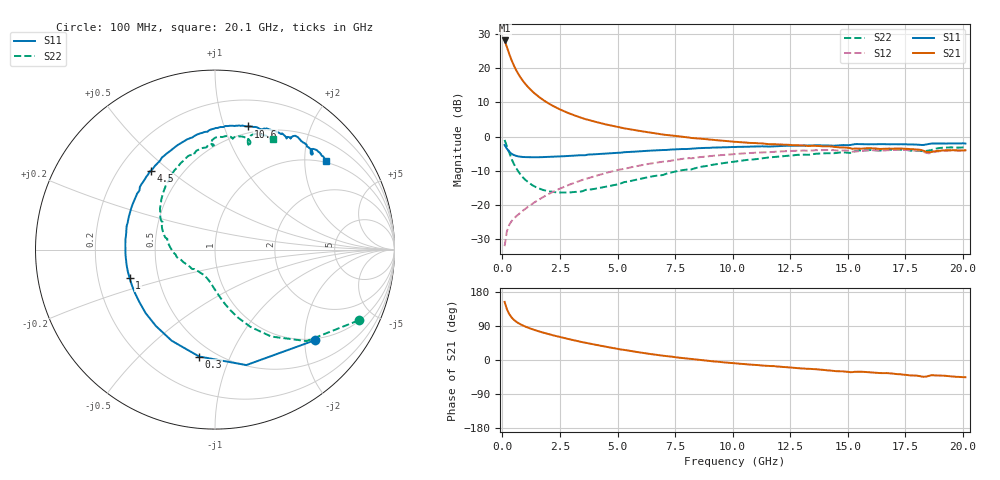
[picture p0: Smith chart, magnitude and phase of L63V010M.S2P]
!  Infineon Technologies AG
! BFR380L3 , PF131585-7, No.6, Th 09.10.01, soldered on pcb-board, measured with PP GSG850
!  Vce=3.0 V,  Ic=10.0 mA
! Common Emitter S-Parameters:  15. November 2001
#  GHz  S  MA  R  50
! f  S11  S21  S12  S22
! GHz  Mag  Ang  Mag  Ang  Mag  Ang  Mag  Ang
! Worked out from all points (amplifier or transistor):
!   201 points, 100 MHz to 20.1 GHz, reference 50 ohm
!   highest |S21| = 28.1 dB at 100 MHz (marker M1)
!   |S21| within 3 dB of that: start of sweep to 253.5 MHz
!   unconditionally stable (mu >= 1): 1.854 GHz to 4.428 GHz
!   at 3.4 GHz: K = 1.03, MAG = 8.2 dB, |S12| = -12.8 dB
!   at 10.1 GHz: K = 0.95, MSG = 1.8 dB, |S12| = -5.1 dB
!   at 20.1 GHz: K = 0.99, MSG = 0.1 dB, |S12| = -4.1 dB
!   S11 on the Smith chart (normalised r, x): 100 MHz: 0.97, -2.25; 300 MHz: 0.41, -0.77; 1 GHz: 0.34, -0.14; 4.5 GHz: 0.33, +0.43; 10.6 GHz: 0.43, +1.21; 20.1 GHz: 0.97, +2.54
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0.1  0.7527 -42.0  25.29 153.3  0.02516 69.2  0.8922 -26.2
0.2  0.6666 -74.8  20.24 133.9  0.04163 58.3  0.721 -45.0
0.3  0.6021 -98.4  16.1 121.2  0.05153 52.1  0.5768 -57.1
0.4  0.5622 -115.4  13.1 112.5  0.05815 49.4  0.4735 -65.4
0.5  0.5383 -127.7  10.94 106.2  0.06334 48.9  0.4 -71.3
0.6  0.5238 -137.7  9.35 101.3  0.06851 49.2  0.3472 -75.9
0.7  0.5126 -145.4  8.157 97.2  0.07316 49.8  0.3073 -79.6
0.8  0.5074 -151.7  7.221 93.8  0.07823 50.8  0.2767 -82.8
1  0.5015 -161.8  5.874 88.2  0.08829 52.6  0.2338 -88.3
1.2  0.5001 -169.7  4.946 83.4  0.09888 54.0  0.2063 -93.0
1.4  0.4994 -176.0  4.278 79.2  0.1098 55.3  0.1873 -97.4
1.6  0.4997 178.4  3.772 75.4  0.121 56.1  0.1746 -101.5
1.9  0.5021 171.2  3.213 70.1  0.1384 56.7  0.1621 -107.5
2.6  0.5154 157.3  2.407 59.2  0.1796 56.3  0.1527 -121.7
3.5  0.5339 142.6  1.847 46.8  0.2346 53.4  0.1601 -137.5
4.5  0.567 129.3  1.503 35.0  0.2946 48.7  0.1858 -156.6
6.8  0.6334 104.2  1.095 12.6  0.4231 34.4  0.2719 168.2
10.1  0.704 78.3  0.8377 -8.6  0.5564 12.8  0.4329 131.4
10.6  0.7104 75.1  0.8172 -11.3  0.5719 9.5  0.456 126.2
13.5  0.7417 60.2  0.7341 -24.2  0.6281 -8.6  0.5545 101.4
16.8  0.7724 47.8  0.6684 -35.0  0.6335 -25.0  0.6423 78.9
20.1  0.7907 38.5  0.632 -45.4  0.6247 -38.8  0.6957 62.1
